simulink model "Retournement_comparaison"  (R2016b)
settings: Solver=ode15s  StartTime=0.0  StopTime=15000  MaxStep=100  RelTol=1e-2  AbsTol=1e-2
undefined symbols (not defined in the file or in its folder): Bague, Bielle, Chassis, deg, kg, m, Manivelle, mm, Moteur, N, Panier_Oeuf, RootGround, RootPart, s, sigbuilder_block, Support_oeufs, Vis
libraries: mblibv1 x42, fl_lib x7, nesl_utility x3, elec_lib x2

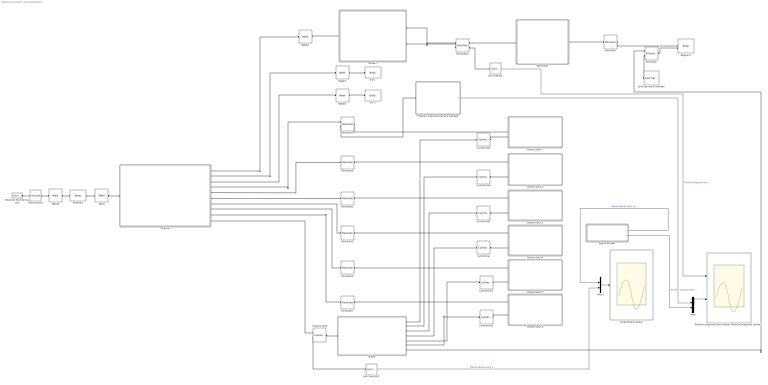
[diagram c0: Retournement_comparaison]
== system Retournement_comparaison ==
  Bague-2 : mblibv1/Bodies/Body  LConnTagsString=CS2|CS3  UpdateFromCAD=on  PMImportedID=Bague-2  DialogClass=MechanicalBodyBlock  Mass=2.57168e-05  MassUnits=kg  InertiaUnits=kg*m^2  Inertia=[4.96681e-11,0,0;0,4.96681e-11,0;0,0,8.21917e-11]  Shape=Cylinder  ShapeDims=[1 1]  ShapeUnits=m  ShapeUse=false  Density=1  DensityUnits=kg/m^3  DensityUse=false  GraphicsMode=GFXFILE  GraphicsFileName=Panier_Oeuf - Bague-2.STL  BodyColorSelMode=COLORPALETTE  BodyColor=[1;0;0]  AttachedToCS=CS1  CG=Right$CG$[0.256568 -0.0741614 -0.063]$WORLD$WORLD$m$[0.897068 0.441893 0;0 0 1;0.441893 -0.897068 0]$3x3 Transform$rad$WORLD$false$Bague-2::CG(AUTOGEN)  WorkingFrames=Right$CS1$[0.256568 -0.0751614 -0.063]$WORLD$WORLD$m$[0.897068 0.441893 0;0 0 1;0.441893 -0.897068 0]$3x3 Transform$rad$WORLD$false$Bague-2::CS1(AUTOGEN)#Left$CS2$[0.256568 -0.0731614 -0.063]$WORLD$WORLD$m$[1 0 0;0 1 0;0 0 1]$3x3 Transform$rad$WORLD$true$Bague-2:-:Manivelle-1::Bague-2(AUTOGEN)#Left$CS3$[0.254568 -0.0731614 -0.065]$WORLD$WORLD$m$[1 0 0;0 1 0;0 0 1]$3x3 Transform$rad$WORLD$true$Bagu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  CGPos=[0.256568 -0.0741614 -0.063]  CGRot=[0.897068 0.441893 0;0 0 1;0.441893 -0.897068 0]  CS0Pos=[]  CS0Rot=[]  CS1Pos=[0.256568 -0.0751614 -0.063]  CS1Rot=[0.897068 0.441893 0;0 0 1;0.441893 -0.897068 0]  CS2Pos=[0.256568 -0.0731614 -0.063]  CS2Rot=[1 0 0;0 1 0;0 0 1]  CS3Pos=[0.254568 -0.0731614 -0.065]  CS3Rot=[1 0 0;0 1 0;0 0 1]  CS4Pos=[]  CS4Rot=[]  CS5Pos=[]  CS5Rot=[]  CS6Pos=[]  CS6Rot=[]  CS7Pos=[]  CS7Rot=[]  CS8Pos=[]  CS8Rot=[]  CS9Pos=[]  CS9Rot=[]  CS10Pos=[]  CS10Rot=[]  CS11Pos=[]  CS11Rot=[]  CS12Pos=[]  CS12Rot=[]  CS13Pos=[]  CS13Rot=[]  CS14Pos=[]  CS14Rot=[]  CS15Pos=[]  CS15Rot=[]  CS16Pos=[]  CS16Rot=[]  CS17Pos=[]  CS17Rot=[]  CS18Pos=[]  CS18Rot=[]  CS19Pos=[]  CS19Rot=[]  CS20Pos=[]  CS20Rot=[]
  Bielle : Subsystem
  Chassis : Subsystem
  "Cinématique bielle " : Scope
  Custom Joint : mblibv1/Joints/Custom Joint  LConnTagsString=__newl0|SA1  RConnTagsString=__newr0  UpdateFromCAD=on  PMImportedID=Bielle-1:-:Chassis-1  NumSAPorts=1  CutJoint=off  MarkAsCut=off  Primitives=prismatic  PrimitiveProps=P1$World$[1,0,0]$prismatic#P2$World$[0,1,0]$prismatic#P3$World$[0,0,1]$prismatic#R1$World$[0,-1,0]$revolute  DialogClass=JointBlock  R1Axis=[0,-1,0]  R2Axis=[]  R3Axis=[]  P1Axis=[1,0,0]  P2Axis=[0,1,0]  P3Axis=[0,0,1]  SAxis=[]
  Cylindrical : mblibv1/Joints/Cylindrical  LConnTagsString=__newl0  RConnTagsString=__newr0  UpdateFromCAD=on  PMImportedID=Bielle-1:-:Support_oeufs-4  NumSAPorts=0  CutJoint=off  MarkAsCut=off  Primitives=prismatic  PrimitiveProps=P1$WORLD$[0,-1,0]$prismatic#R1$WORLD$[0,-1,0]$revolute  DialogClass=JointBlock  P1Axis=[0,-1,0]  R1Axis=[0,-1,0]
  Cylindrical1 : mblibv1/Joints/Cylindrical  LConnTagsString=__newl0  RConnTagsString=__newr0  UpdateFromCAD=on  PMImportedID=Bielle-1:-:Support_oeufs-3  NumSAPorts=0  CutJoint=off  MarkAsCut=off  Primitives=prismatic  PrimitiveProps=P1$WORLD$[0,-1,0]$prismatic#R1$WORLD$[0,-1,0]$revolute  DialogClass=JointBlock  P1Axis=[0,-1,0]  R1Axis=[0,-1,0]
  Cylindrical2 : mblibv1/Joints/Cylindrical  LConnTagsString=__newl0  RConnTagsString=__newr0  UpdateFromCAD=on  PMImportedID=Bielle-1:-:Support_oeufs-5  NumSAPorts=0  CutJoint=off  MarkAsCut=off  Primitives=prismatic  PrimitiveProps=P1$WORLD$[0,-1,0]$prismatic#R1$WORLD$[0,-1,0]$revolute  DialogClass=JointBlock  P1Axis=[0,-1,0]  R1Axis=[0,-1,0]
  Cylindrical3 : mblibv1/Joints/Cylindrical  LConnTagsString=__newl0  RConnTagsString=__newr0  UpdateFromCAD=on  PMImportedID=Bielle-1:-:Support_oeufs-6  NumSAPorts=0  CutJoint=off  MarkAsCut=off  Primitives=prismatic  PrimitiveProps=P1$WORLD$[0,-1,0]$prismatic#R1$WORLD$[0,-1,0]$revolute  DialogClass=JointBlock  P1Axis=[0,-1,0]  R1Axis=[0,-1,0]
  Cylindrical4 : mblibv1/Joints/Cylindrical  LConnTagsString=__newl0  RConnTagsString=__newr0  UpdateFromCAD=on  PMImportedID=Bielle-1:-:Support_oeufs-2  NumSAPorts=0  CutJoint=off  MarkAsCut=off  Primitives=prismatic  PrimitiveProps=P1$WORLD$[0,-1,0]$prismatic#R1$WORLD$[0,-1,0]$revolute  DialogClass=JointBlock  P1Axis=[0,-1,0]  R1Axis=[0,-1,0]
  Cylindrical5 : mblibv1/Joints/Cylindrical  LConnTagsString=__newl0  RConnTagsString=__newr0  UpdateFromCAD=on  PMImportedID=Bielle-1:-:Support_oeufs-1  NumSAPorts=0  CutJoint=off  MarkAsCut=off  Primitives=prismatic  PrimitiveProps=P1$WORLD$[0,-1,0]$prismatic#R1$WORLD$[0,-1,0]$revolute  DialogClass=JointBlock  P1Axis=[0,-1,0]  R1Axis=[0,-1,0]
  Joint Sensor : mblibv1/Sensors &  Actuators/Joint Sensor  UpdateFromCAD=off  PhysicalDomain=Mechanical  PortType=blob  Muxed=off  Pose=off  Angle=on  AngleUnits=deg  ArcVelocity=off  ArcVelocityUnits=rpm  ArcAcceleration=off  ArcAccelerationUnits=deg/s^2  CoordPosition=on  CoordPositionUnits=m  Velocity=off  VelocityUnits=m/s  Acceleration=off  AccelerationUnits=m/s^2  Quaternion=on  QuaternionDT=off  QuaternionDDT=off  QuaternionUnits=off  OutputVector=[1]  ActiveIO=on  Width=1  DialogClass=MechanicalSensorBlock  Primitive=R1  Force=off  ForceUnits=N  Torque=off  TorqueUnits=N*m  ReferenceFrame=Absolute (World)  ReactionSensedSide=Follower  ReactionReferenceFrame=Absolute (World)  ReactionForce=off  ReactionForceUnits=N  ReactionMoment=off  ReactionMomentUnits=N*m
  Joint Sensor3 : mblibv1/Sensors &  Actuators/Joint Sensor  UpdateFromCAD=off  PhysicalDomain=Mechanical  PortType=blob  Muxed=off  Pose=off  Angle=on  AngleUnits=deg  ArcVelocity=off  ArcVelocityUnits=rpm  ArcAcceleration=off  ArcAccelerationUnits=deg/s^2  CoordPosition=on  CoordPositionUnits=mm  Velocity=off  VelocityUnits=mm/s  Acceleration=off  AccelerationUnits=m/s^2  Quaternion=on  QuaternionDT=off  QuaternionDDT=off  QuaternionUnits=off  OutputVector=[1]  ActiveIO=on  Width=1  DialogClass=MechanicalSensorBlock  Primitive=P1  Force=off  ForceUnits=N  Torque=off  TorqueUnits=N*m  ReferenceFrame=Absolute (World)  ReactionSensedSide=Follower  ReactionReferenceFrame=Absolute (World)  ReactionForce=off  ReactionForceUnits=N  ReactionMoment=off  ReactionMomentUnits=N*m
  Joint Spring & Damper : mblibv1/Force  Elements/Joint Spring & Damper  UpdateFromCAD=off  DialogClass=JointSpringDamper  JFEParameters=P1$true$0$0.1$0$m$m/s$N$deg$deg/s$N*m#P2$false$0$0$0$m$m/s$N$deg$deg/s$N*m#P3$false$0$0$0$m$m/s$N$deg$deg/s$N*m#R1$false$0$0$0$m$m/s$N$deg$deg/s$N*m#R2$false$0$0$0$m$m/s$N$deg$deg/s$N*m#R3$false$0$0$0$m$m/s$N$deg$deg/s$N*m#S$false$0$0$0$m$m/s$N$deg$deg/s$N*m
  Machine Environment1 : mblibv1/Bodies/Machine Environment  PortType=env  PhysicalDomain=Mechanical  DialogTemplateClass=MECH.MachineEnvironment  SyncWhenCopied=off  Gravity=[0 -9.81 0]  GravityUnits=m/s^2  GravityAsSignal=off  Dimensionality=Auto-detect  AnalysisType=Forward dynamics  LinearAssemblyTolerance=1e-3  LinearAssemblyToleranceUnits=m  AngularAssemblyTolerance=1e-3  AngularAssemblyToleranceUnits=rad  ConstraintSolverType=Tolerancing  ConstraintRelTolerance=1e-3  ConstraintAbsTolerance=1e-3  UseRobustSingularityHandling=off  RedundancyAnalysisToleranceType=Specify tolerance  RedundancyAnalysisTolerance=1e-5  StatePerturbationType=Fixed  PerturbationSize=1e-5  VisualizeMachine=on  BodyVisualizationType=Use model default body geometries  BodyColorSelMode=Use model default  DefaultBodyColor=[1 0 0]
  Manivelle : Subsystem
  Moteur : Subsystem
  Mux : Mux  Inputs=2
  Mux1 : Mux  Inputs=2
  Panier Oeuf 1 : Subsystem
  Panier Oeuf 2 : Subsystem
  Panier Oeuf 3 : Subsystem
  Panier Oeuf 4 : Subsystem
  Panier Oeuf 5 : Subsystem
  Panier Oeuf 6 : Subsystem
  Position angulaire Paniers simulée : Subsystem
  "Position angulaire axe moteur Position angulaire paniers " : Scope  NumInputPorts=2
  Prismatic : mblibv1/Joints/Prismatic  LConnTagsString=__newl0|SA1  RConnTagsString=__newr0  UpdateFromCAD=on  PMImportedID=Bague-2:-:Bielle-1  NumSAPorts=1  CutJoint=off  MarkAsCut=off  Primitives=prismatic  PrimitiveProps=P1$World$[0,0,1]$prismatic  DialogClass=JointBlock  P1Axis=[0,0,1]
  Revolute : mblibv1/Joints/Revolute  LConnTagsString=__newl0  RConnTagsString=__newr0  UpdateFromCAD=on  PMImportedID=Bague-2:-:Manivelle-1  NumSAPorts=0  CutJoint=off  MarkAsCut=off  Primitives=prismatic  PrimitiveProps=R1$WORLD$[0,1,0]$revolute  DialogClass=JointBlock  R1Axis=[0,1,0]
  Revolute1 : mblibv1/Joints/Revolute  LConnTagsString=__newl0  RConnTagsString=__newr0  UpdateFromCAD=on  PMImportedID=Chassis-1:-:Support_oeufs-4  NumSAPorts=0  CutJoint=off  MarkAsCut=off  Primitives=prismatic  PrimitiveProps=R1$WORLD$[0,-1,0]$revolute  DialogClass=JointBlock  R1Axis=[0,-1,0]
  Revolute2 : mblibv1/Joints/Revolute  LConnTagsString=__newl0  RConnTagsString=__newr0  UpdateFromCAD=on  PMImportedID=Chassis-1:-:Support_oeufs-3  NumSAPorts=0  CutJoint=off  MarkAsCut=off  Primitives=prismatic  PrimitiveProps=R1$WORLD$[0,-1,0]$revolute  DialogClass=JointBlock  R1Axis=[0,-1,0]
  Revolute3 : mblibv1/Joints/Revolute  LConnTagsString=__newl0|SA1  RConnTagsString=__newr0|SA1  UpdateFromCAD=on  PMImportedID=Manivelle-1:-:Moteur-1  NumSAPorts=2  CutJoint=off  MarkAsCut=off  Primitives=prismatic  PrimitiveProps=R1$World$[0,-1,0]$revolute  DialogClass=JointBlock  R1Axis=[0,-1,0]
  Revolute5 : mblibv1/Joints/Revolute  LConnTagsString=__newl0  RConnTagsString=__newr0  UpdateFromCAD=on  PMImportedID=Chassis-1:-:Support_oeufs-5  NumSAPorts=0  CutJoint=off  MarkAsCut=off  Primitives=prismatic  PrimitiveProps=R1$WORLD$[0,-1,0]$revolute  DialogClass=JointBlock  R1Axis=[0,-1,0]
  Revolute7 : mblibv1/Joints/Revolute  LConnTagsString=__newl0  RConnTagsString=__newr0  UpdateFromCAD=on  PMImportedID=Chassis-1:-:Support_oeufs-6  NumSAPorts=0  CutJoint=off  MarkAsCut=off  Primitives=prismatic  PrimitiveProps=R1$WORLD$[0,-1,0]$revolute  DialogClass=JointBlock  R1Axis=[0,-1,0]
  Revolute8 : mblibv1/Joints/Revolute  LConnTagsString=__newl0  RConnTagsString=__newr0  UpdateFromCAD=on  PMImportedID=Chassis-1:-:Support_oeufs-2  NumSAPorts=0  CutJoint=off  MarkAsCut=off  Primitives=prismatic  PrimitiveProps=R1$WORLD$[0,-1,0]$revolute  DialogClass=JointBlock  R1Axis=[0,-1,0]
  Revolute9 : mblibv1/Joints/Revolute  LConnTagsString=__newl0|SA1  RConnTagsString=__newr0  UpdateFromCAD=on  PMImportedID=Chassis-1:-:Support_oeufs-1  NumSAPorts=1  CutJoint=off  MarkAsCut=off  Primitives=prismatic  PrimitiveProps=R1$World$[0,-1,0]$revolute  DialogClass=JointBlock  R1Axis=[0,-1,0]
  RootGround : mblibv1/Bodies/Ground  UpdateFromCAD=on  PMImportedID=RootGround  LeftPortType=env  RightPortType=workingframe  PhysicalDomain=Mechanical  DialogClass=GroundBlock  CoordPosition=[0.0985288,0.0399076,-0.023573]  CoordPositionUnits=m  StateVectorMgrId=-1  MachineId=[0 0]  ShowEnvPort=on  ParameterChecksum=[42814579, 2142450646, 2016383780, 4272844323]  TopologyChecksum=[3713097820, 1283573318, 1879926558, 343871556]
  RootPart : mblibv1/Bodies/Body  LConnTagsString=CS3  RConnTagsString=CS2  UpdateFromCAD=on  PMImportedID=Panier_Oeuf/RootPart  DialogClass=MechanicalBodyBlock  Mass=0  MassUnits=kg  InertiaUnits=kg*m^2  Inertia=[0,0,0;0,0,0;0,0,0]  Shape=Cylinder  ShapeDims=[1 1]  ShapeUnits=m  ShapeUse=false  Density=1  DensityUnits=kg/m^3  DensityUse=false  GraphicsMode=MACHINE_DEFAULT  BodyColorSelMode=MACHINE_DEFAULT  BodyColor=[1;0;0]  AttachedToCS=CS1  CG=Right$CG$[0.0985288 0.0399076 -0.023573]$WORLD$WORLD$m$[1 0 0;0 1 0;0 0 1]$3x3 Transform$rad$WORLD$false$Panier_Oeuf/RootPart::CG(AUTOGEN)  WorkingFrames=Right$CS1$[0 0 0]$WORLD$WORLD$m$[1 0 0;0 1 0;0 0 1]$3x3 Transform$rad$WORLD$false$Panier_Oeuf/RootPart::CS1(AUTOGEN)#Right$CS2$[0.0811984 0.0557636 -0.00887792]$WORLD$WORLD$m$[1 0 0;0 1 0;0 0 1]$3x3 Transform$rad$WORLD$true$Chassis-1:-:Panier_Oeuf/RootPart::Panier_Oeuf/RootPart(AUTOGEN)#Left$CS3$[0.0985288 0.0399076 -0.023573]$WORLD$WORLD$m$[1 0 0;0 1 0;0 0 1]$3x3 Transform$rad$WORLD$true$Panier_O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  CGPos=[0.0985288 0.0399076 -0.023573]  CGRot=[1 0 0;0 1 0;0 0 1]  CS0Pos=[]  CS0Rot=[]  CS1Pos=[0 0 0]  CS1Rot=[1 0 0;0 1 0;0 0 1]  CS2Pos=[0.0811984 0.0557636 -0.00887792]  CS2Rot=[1 0 0;0 1 0;0 0 1]  CS3Pos=[0.0985288 0.0399076 -0.023573]  CS3Rot=[1 0 0;0 1 0;0 0 1]  CS4Pos=[]  CS4Rot=[]  CS5Pos=[]  CS5Rot=[]  CS6Pos=[]  CS6Rot=[]  CS7Pos=[]  CS7Rot=[]  CS8Pos=[]  CS8Rot=[]  CS9Pos=[]  CS9Rot=[]  CS10Pos=[]  CS10Rot=[]  CS11Pos=[]  CS11Rot=[]  CS12Pos=[]  CS12Rot=[]  CS13Pos=[]  CS13Rot=[]  CS14Pos=[]  CS14Rot=[]  CS15Pos=[]  CS15Rot=[]  CS16Pos=[]  CS16Rot=[]  CS17Pos=[]  CS17Rot=[]  CS18Pos=[]  CS18Rot=[]  CS19Pos=[]  CS19Rot=[]  CS20Pos=[]  CS20Rot=[]
  Signal Builder : Subsystem  Tag=STV Subsys  LoadFcn=sigbuilder_block('load');  StartFcn=sigbuilder_block('start');  StopFcn=sigbuilder_block('stop');  ClipboardFcn=sigbuilder_block('clipboard');
  Vis-1 : mblibv1/Bodies/Body  LConnTagsString=CS2  UpdateFromCAD=on  PMImportedID=Vis-1  DialogClass=MechanicalBodyBlock  Mass=0.000201069  MassUnits=kg  InertiaUnits=kg*m^2  Inertia=[1.44008e-09,0,0;0,1.44008e-09,0;0,0,1.17522e-09]  Shape=Cylinder  ShapeDims=[1 1]  ShapeUnits=m  ShapeUse=false  Density=1  DensityUnits=kg/m^3  DensityUse=false  GraphicsMode=GFXFILE  GraphicsFileName=Panier_Oeuf - Vis-1.STL  BodyColorSelMode=COLORPALETTE  BodyColor=[0.792157;0.819608;0.933333]  AttachedToCS=CS1  CG=Right$CG$[0.274549 -0.0683931 -0.022]$WORLD$WORLD$m$[-0.990019 -0.140935 0;0 0 1;-0.140935 0.990019 0]$3x3 Transform$rad$WORLD$false$Vis-1::CG(AUTOGEN)  WorkingFrames=Right$CS1$[0.274549 -0.0681614 -0.022]$WORLD$WORLD$m$[-0.990019 -0.140935 0;0 0 1;-0.140935 0.990019 0]$3x3 Transform$rad$WORLD$false$Vis-1::CS1(AUTOGEN)#Left$CS2$[0.274549 -0.0681614 -0.022]$WORLD$WORLD$m$[1 0 0;0 1 0;0 0 1]$3x3 Transform$rad$WORLD$true$Chassis-1:-:Vis-1::Vis-1(AUTOGEN)  CGPos=[0.274549 -0.0683931 -0.022]  CGRot=[-0.990019 -0.140935 0;0 0 1;-0.140935 0.990019 0]  CS0Pos=[]  CS0Rot=[]  CS1Pos=[0.274549 -0.0681614 -0.022]  CS1Rot=[-0.990019 -0.140935 0;0 0 1;-0.140935 0.990019 0]  CS2Pos=[0.274549 -0.0681614 -0.022]  CS2Rot=[1 0 0;0 1 0;0 0 1]  CS3Pos=[]  CS3Rot=[]  CS4Pos=[]  CS4Rot=[]  CS5Pos=[]  CS5Rot=[]  CS6Pos=[]  CS6Rot=[]  CS7Pos=[]  CS7Rot=[]  CS8Pos=[]  CS8Rot=[]  CS9Pos=[]  CS9Rot=[]  CS10Pos=[]  CS10Rot=[]  CS11Pos=[]  CS11Rot=[]  CS12Pos=[]  CS12Rot=[]  CS13Pos=[]  CS13Rot=[]  CS14Pos=[]  CS14Rot=[]  CS15Pos=[]  CS15Rot=[]  CS16Pos=[]  CS16Rot=[]  CS17Pos=[]  CS17Rot=[]  CS18Pos=[]  CS18Rot=[]  CS19Pos=[]  CS19Rot=[]  CS20Pos=[]  CS20Rot=[]
  Vis-2 : mblibv1/Bodies/Body  LConnTagsString=CS2  UpdateFromCAD=on  PMImportedID=Vis-2  DialogClass=MechanicalBodyBlock  Mass=0.000201069  MassUnits=kg  InertiaUnits=kg*m^2  Inertia=[1.44008e-09,0,0;0,1.44008e-09,0;0,0,1.17522e-09]  Shape=Cylinder  ShapeDims=[1 1]  ShapeUnits=m  ShapeUse=false  Density=1  DensityUnits=kg/m^3  DensityUse=false  GraphicsMode=GFXFILE  GraphicsFileName=Panier_Oeuf - Vis-2.STL  BodyColorSelMode=COLORPALETTE  BodyColor=[0.792157;0.819608;0.933333]  AttachedToCS=CS1  CG=Right$CG$[0.262549 -0.0683931 -0.022]$WORLD$WORLD$m$[-0.990019 -0.140935 0;0 0 1;-0.140935 0.990019 0]$3x3 Transform$rad$WORLD$false$Vis-2::CG(AUTOGEN)  WorkingFrames=Right$CS1$[0.262549 -0.0681614 -0.022]$WORLD$WORLD$m$[-0.990019 -0.140935 0;0 0 1;-0.140935 0.990019 0]$3x3 Transform$rad$WORLD$false$Vis-2::CS1(AUTOGEN)#Left$CS2$[0.262549 -0.0681614 -0.022]$WORLD$WORLD$m$[1 0 0;0 1 0;0 0 1]$3x3 Transform$rad$WORLD$true$Chassis-1:-:Vis-2::Vis-2(AUTOGEN)  CGPos=[0.262549 -0.0683931 -0.022]  CGRot=[-0.990019 -0.140935 0;0 0 1;-0.140935 0.990019 0]  CS0Pos=[]  CS0Rot=[]  CS1Pos=[0.262549 -0.0681614 -0.022]  CS1Rot=[-0.990019 -0.140935 0;0 0 1;-0.140935 0.990019 0]  CS2Pos=[0.262549 -0.0681614 -0.022]  CS2Rot=[1 0 0;0 1 0;0 0 1]  CS3Pos=[]  CS3Rot=[]  CS4Pos=[]  CS4Rot=[]  CS5Pos=[]  CS5Rot=[]  CS6Pos=[]  CS6Rot=[]  CS7Pos=[]  CS7Rot=[]  CS8Pos=[]  CS8Rot=[]  CS9Pos=[]  CS9Rot=[]  CS10Pos=[]  CS10Rot=[]  CS11Pos=[]  CS11Rot=[]  CS12Pos=[]  CS12Rot=[]  CS13Pos=[]  CS13Rot=[]  CS14Pos=[]  CS14Rot=[]  CS15Pos=[]  CS15Rot=[]  CS16Pos=[]  CS16Rot=[]  CS17Pos=[]  CS17Rot=[]  CS18Pos=[]  CS18Rot=[]  CS19Pos=[]  CS19Rot=[]  CS20Pos=[]  CS20Rot=[]
  Weld : mblibv1/Joints/Weld  LConnTagsString=__newl0  RConnTagsString=__newr0  UpdateFromCAD=on  PMImportedID=Chassis-1:-:Panier_Oeuf/RootPart  NumSAPorts=0  CutJoint=off  MarkAsCut=off  Primitives=weld  PrimitiveProps=W$WORLD$[0.57735,0.57735,0.57735]$weld  DialogClass=JointBlock  WAxis=[0.57735,0.57735,0.57735]
  Weld1 : mblibv1/Joints/Weld  LConnTagsString=__newl0  RConnTagsString=__newr0  UpdateFromCAD=on  PMImportedID=Chassis-1:-:Moteur-1  NumSAPorts=0  CutJoint=off  MarkAsCut=off  Primitives=weld  PrimitiveProps=W$WORLD$[0.57735,0.57735,0.57735]$weld  DialogClass=JointBlock  WAxis=[0.57735,0.57735,0.57735]
  Weld2 : mblibv1/Joints/Weld  LConnTagsString=__newl0  RConnTagsString=__newr0  UpdateFromCAD=on  PMImportedID=Panier_Oeuf/RootPart:-:RootGround  NumSAPorts=0  CutJoint=off  MarkAsCut=off  Primitives=weld  PrimitiveProps=W$WORLD$[0.57735,0.57735,0.57735]$weld  DialogClass=JointBlock  WAxis=[0.57735,0.57735,0.57735]
  Weld3 : mblibv1/Joints/Weld  LConnTagsString=__newl0  RConnTagsString=__newr0  UpdateFromCAD=on  NumSAPorts=0  CutJoint=off  MarkAsCut=off  Primitives=weld  PrimitiveProps=W$WORLD$[0.57735,0.57735,0.57735]$weld  DialogClass=JointBlock  WAxis=[0.57735,0.57735,0.57735]
  Weld4 : mblibv1/Joints/Weld  LConnTagsString=__newl0  RConnTagsString=__newr0  UpdateFromCAD=on  NumSAPorts=0  CutJoint=off  MarkAsCut=off  Primitives=weld  PrimitiveProps=W$WORLD$[0.57735,0.57735,0.57735]$weld  DialogClass=JointBlock  WAxis=[0.57735,0.57735,0.57735]
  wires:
  Joint Sensor/1 -> "Position angulaire axe moteur Position angulaire paniers "/1  "Position angulaire axe moteur simulée"
  Joint Sensor3/1 -> Mux1/2  "Position Bielle axe X simulée"
  Signal Builder/2(Position Ang Paniers) -> Mux/2  "Position angulaire Paniers mesurée"
  Mux/1 -> "Position angulaire axe moteur Position angulaire paniers "/2
  Mux1/1 -> "Cinématique bielle "/1
  Signal Builder/1(Position Bielle Axe X) -> Mux1/1  "Position Bielle axe X mesurée"
  Position angulaire Paniers simulée/1(Out1) -> Mux/1
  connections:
  RootPart/RConn1 -- Weld/LConn1
  Revolute/RConn1 -- Bague-2/LConn1
  Prismatic/RConn1 -- Bague-2/LConn2
  Panier Oeuf 4/LConn1 -- Revolute1/RConn1
  Panier Oeuf 4/LConn2 -- Cylindrical/RConn1
  Panier Oeuf 3/LConn1 -- Revolute2/RConn1
  Panier Oeuf 3/LConn2 -- Cylindrical1/RConn1
  Weld4/RConn1 -- Vis-2/LConn1
  Panier Oeuf 5/LConn1 -- Revolute5/RConn1
  Panier Oeuf 5/LConn2 -- Cylindrical2/RConn1
  Weld3/RConn1 -- Vis-1/LConn1
  Panier Oeuf 6/LConn1 -- Revolute7/RConn1
  Panier Oeuf 2/LConn1 -- Revolute8/RConn1
  Revolute9/RConn1 -- Panier Oeuf 1/LConn1
  Cylindrical3/RConn1 -- Panier Oeuf 6/LConn2
  Panier Oeuf 2/LConn2 -- Cylindrical4/RConn1
  Cylindrical5/RConn1 -- Panier Oeuf 1/LConn2
  RootGround/RConn1 -- Weld2/LConn1
  Weld2/RConn1 -- RootPart/LConn1
  Machine Environment1/RConn1 -- RootGround/LConn1
  Joint Spring & Damper/LConn1 -- Prismatic/LConn2
  Moteur/RConn1 -- Revolute3/LConn1
  Weld1/RConn1 -- Moteur/LConn1
  Revolute3/LConn2 -- Moteur/RConn2
  Manivelle/LConn1 -- Revolute3/RConn1
  Manivelle/RConn1 -- Revolute/LConn1
  Prismatic/LConn1 -- Bielle/RConn7
  Bielle/RConn1 -- Cylindrical5/LConn1
  Bielle/RConn2 -- Cylindrical4/LConn1
  Bielle/RConn3 -- Cylindrical1/LConn1
  Bielle/RConn4 -- Cylindrical/LConn1
  Cylindrical2/LConn1 -- Bielle/RConn5
  Bielle/RConn6 -- Cylindrical3/LConn1
  Custom Joint/RConn1 -- Bielle/LConn1
  Weld1/LConn1 -- Chassis/RConn1
  Weld3/LConn1 -- Chassis/RConn2
  Weld4/LConn1 -- Chassis/RConn3
  Revolute9/LConn1 -- Chassis/RConn4
  Revolute8/LConn1 -- Chassis/RConn5
  Revolute2/LConn1 -- Chassis/RConn6
  Revolute1/LConn1 -- Chassis/RConn7
  Weld/RConn1 -- Chassis/LConn1
  Revolute5/LConn1 -- Chassis/RConn8
  Revolute7/LConn1 -- Chassis/RConn9
  Custom Joint/LConn1 -- Chassis/RConn10
  Revolute3/RConn2 -- Joint Sensor/LConn1
  Custom Joint/LConn2 -- Joint Sensor3/LConn1
  Position angulaire Paniers simulée/LConn1 -- Revolute9/LConn2

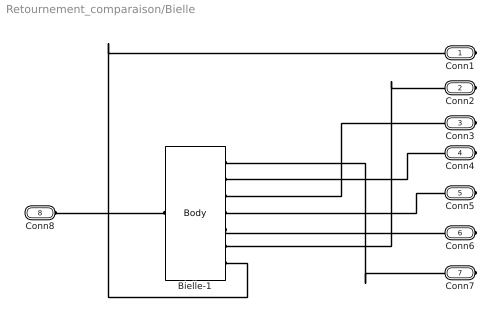
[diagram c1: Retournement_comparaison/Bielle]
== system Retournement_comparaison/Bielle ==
  Bielle-1 : mblibv1/Bodies/Body  LConnTagsString=CS6  RConnTagsString=CS2|CS3|CS4|CS5|CS7|CS8|CS9  UpdateFromCAD=on  PMImportedID=Bielle-1  DialogClass=MechanicalBodyBlock  Mass=0.0183422  MassUnits=kg  InertiaUnits=kg*m^2  Inertia=[1.02402e-06,1.48492e-06,-1.23168e-06;1.48492e-06,0.000206355,2.24204e-08;-1.23168e-06,2.24204e-08,0.00020726]  Shape=Cylinder  ShapeDims=[1 1]  ShapeUnits=m  ShapeUse=false  Density=1  DensityUnits=kg/m^3  DensityUse=false  GraphicsMode=GFXFILE  GraphicsFileName=Panier_Oeuf - Bielle-1.STL  BodyColorSelMode=COLORPALETTE  BodyColor=[1;1;0]  AttachedToCS=CS1  CG=Right$CG$[0.125761 -0.080148 -0.0505953]$WORLD$WORLD$m$[-1 0 0;0 0 -1;0 -1 0]$3x3 Transform$rad$WORLD$false$Bielle-1::CG(AUTOGEN)  WorkingFrames=Right$CS1$[0.231882 -0.0791614 -0.0940911]$WORLD$WORLD$m$[-1 0 0;0 0 -1;0 -1 0]$3x3 Transform$rad$WORLD$false$Bielle-1::CS1(AUTOGEN)#Right$CS2$[0.254568 -0.0731614 -0.0309764]$WORLD$WORLD$m$[1 0 0;0 1 0;0 0 1]$3x3 Transform$rad$WORLD$true$Bague-2:-:Bielle-1::Bielle-1(AUTOGEN)#Right$CS3$[0.100768 -0.0791614 -0.0499764]$WORLD$WORLD$m$[1 0 0;0 1 0;0 0 1]$3x3 Transform$rad$WORLD$true$Bielle-1:-:Suppor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  CGPos=[0.125761 -0.080148 -0.0505953]  CGRot=[-1 0 0;0 0 -1;0 -1 0]  CS0Pos=[]  CS0Rot=[]  CS1Pos=[0.231882 -0.0791614 -0.0940911]  CS1Rot=[-1 0 0;0 0 -1;0 -1 0]  CS2Pos=[0.254568 -0.0731614 -0.0309764]  CS2Rot=[1 0 0;0 1 0;0 0 1]  CS3Pos=[0.100768 -0.0791614 -0.0499764]  CS3Rot=[1 0 0;0 1 0;0 0 1]  CS4Pos=[0.046368 -0.0791614 -0.0499764]  CS4Rot=[1 0 0;0 1 0;0 0 1]  CS5Pos=[0.155168 -0.0791614 -0.0499764]  CS5Rot=[1 0 0;0 1 0;0 0 1]  CS6Pos=[0.104549 -0.0681614 0.003]  CS6Rot=[1 0 0;0 1 0;0 0 1]  CS7Pos=[0.209568 -0.0791614 -0.0499764]  CS7Rot=[1 0 0;0 1 0;0 0 1]  CS8Pos=[-0.00803199 -0.0791614 -0.0499764]  CS8Rot=[1 0 0;0 1 0;0 0 1]  CS9Pos=[-0.062432 -0.0791614 -0.0499764]  CS9Rot=[1 0 0;0 1 0;0 0 1]  CS10Pos=[]  CS10Rot=[]  CS11Pos=[]  CS11Rot=[]  CS12Pos=[]  CS12Rot=[]  CS13Pos=[]  CS13Rot=[]  CS14Pos=[]  CS14Rot=[]  CS15Pos=[]  CS15Rot=[]  CS16Pos=[]  CS16Rot=[]  CS17Pos=[]  CS17Rot=[]  CS18Pos=[]  CS18Rot=[]  CS19Pos=[]  CS19Rot=[]  CS20Pos=[]  CS20Rot=[]
  Conn1 : PMIOPort  Port=1  Side=Right
  Conn2 : PMIOPort  Port=2  Side=Right
  Conn3 : PMIOPort  Port=3  Side=Right
  Conn4 : PMIOPort  Port=4  Side=Right
  Conn5 : PMIOPort  Port=5  Side=Right
  Conn6 : PMIOPort  Port=6  Side=Right
  Conn7 : PMIOPort  Port=7  Side=Right
  Conn8 : PMIOPort  Port=8  Side=Left
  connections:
  Bielle-1/RConn4 -- Conn5/RConn1
  Conn8/RConn1 -- Bielle-1/LConn1
  Bielle-1/RConn7 -- Conn1/RConn1
  Bielle-1/RConn5 -- Conn6/RConn1
  Bielle-1/RConn6 -- Conn2/RConn1
  Bielle-1/RConn1 -- Conn7/RConn1
  Bielle-1/RConn2 -- Conn4/RConn1
  Bielle-1/RConn3 -- Conn3/RConn1

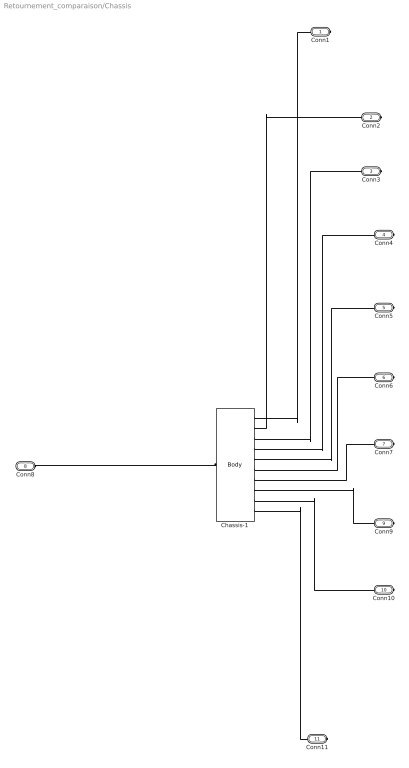
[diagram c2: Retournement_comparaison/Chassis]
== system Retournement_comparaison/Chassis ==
  Chassis-1 : mblibv1/Bodies/Body  LConnTagsString=CS2  RConnTagsString=CS3|CS4|CS5|CS6|CS7|CS8|CS9|CS10|CS11|CS12  UpdateFromCAD=on  PMImportedID=Chassis-1  DialogClass=MechanicalBodyBlock  Mass=0.187115  MassUnits=kg  InertiaUnits=kg*m^2  Inertia=[0.00212227,3.19267e-05,-2.28618e-06;3.19267e-05,0.00278137,7.43577e-06;-2.28618e-06,7.43577e-06,0.00485618]  Shape=Cylinder  ShapeDims=[1 1]  ShapeUnits=m  ShapeUse=false  Density=1  DensityUnits=kg/m^3  DensityUse=false  GraphicsMode=GFXFILE  GraphicsFileName=Panier_Oeuf - Chassis-1.STL  BodyColorSelMode=COLORPALETTE  BodyColor=[0 1 0]  AttachedToCS=CS1  CG=Right$CG$[0.0811984 0.0557636 -0.00887792]$WORLD$WORLD$m$[1 0 0;0 1 0;0 0 1]$3x3 Transform$rad$WORLD$false$Chassis-1::CG(AUTOGEN)  WorkingFrames=Right$CS1$[0 0 0]$WORLD$WORLD$m$[1 0 0;0 1 0;0 0 1]$3x3 Transform$rad$WORLD$false$Chassis-1::CS1(AUTOGEN)#Left$CS2$[0.0811984 0.0557636 -0.00887792]$WORLD$WORLD$m$[1 0 0;0 1 0;0 0 1]$3x3 Transform$rad$WORLD$true$Chassis-1:-:Panier_Oeuf/RootPart::Chassis-1(AUTOGEN)#Right$CS3$[0.282549 -0.0651614 0.003]$WORLD$WORLD$m$[1 0 0;0 1 0;0 0 1]$3x3 Transform$rad$WORLD$true$Chassis-1:-:Support_oeufs-4::Chass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  CGPos=[0.0811984 0.0557636 -0.00887792]  CGRot=[1 0 0;0 1 0;0 0 1]  CS0Pos=[]  CS0Rot=[]  CS1Pos=[0 0 0]  CS1Rot=[1 0 0;0 1 0;0 0 1]  CS2Pos=[0.0811984 0.0557636 -0.00887792]  CS2Rot=[1 0 0;0 1 0;0 0 1]  CS3Pos=[0.282549 -0.0651614 0.003]  CS3Rot=[1 0 0;0 1 0;0 0 1]  CS4Pos=[0.274549 -0.0681614 -0.022]  CS4Rot=[1 0 0;0 1 0;0 0 1]  CS5Pos=[0.262549 -0.0681614 -0.022]  CS5Rot=[1 0 0;0 1 0;0 0 1]  CS6Pos=[-0.0634506 0.192839 -0.028]  CS6Rot=[1 0 0;0 1 0;0 0 1]  CS7Pos=[-0.00905056 -0.0651614 -0.028]  CS7Rot=[1 0 0;0 1 0;0 0 1]  CS8Pos=[0.0453494 0.192839 -0.028]  CS8Rot=[1 0 0;0 1 0;0 0 1]  CS9Pos=[0.0997494 0.192839 -0.028]  CS9Rot=[1 0 0;0 1 0;0 0 1]  CS10Pos=[0.154149 0.192839 -0.028]  CS10Rot=[1 0 0;0 1 0;0 0 1]  CS11Pos=[0.208549 0.192839 -0.028]  CS11Rot=[1 0 0;0 1 0;0 0 1]  CS12Pos=[0.104549 -0.0681614 0.003]  CS12Rot=[1 0 0;0 1 0;0 0 1]  CS13Pos=[]  CS13Rot=[]  CS14Pos=[]  CS14Rot=[]  CS15Pos=[]  CS15Rot=[]  CS16Pos=[]  CS16Rot=[]  CS17Pos=[]  CS17Rot=[]  CS18Pos=[]  CS18Rot=[]  CS19Pos=[]  CS19Rot=[]  CS20Pos=[]  CS20Rot=[]
  Conn1 : PMIOPort  Port=1  Side=Right
  Conn2 : PMIOPort  Port=2  Side=Right
  Conn3 : PMIOPort  Port=3  Side=Right
  Conn4 : PMIOPort  Port=4  Side=Right
  Conn5 : PMIOPort  Port=5  Side=Right
  Conn6 : PMIOPort  Port=6  Side=Right
  Conn7 : PMIOPort  Port=7  Side=Right
  Conn8 : PMIOPort  Port=8  Side=Left
  Conn9 : PMIOPort  Port=9  Side=Right
  Conn10 : PMIOPort  Port=10  Side=Right
  Conn11 : PMIOPort  Port=11  Side=Right
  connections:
  Chassis-1/RConn2 -- Conn2/RConn1
  Conn5/RConn1 -- Chassis-1/RConn5
  Conn10/RConn1 -- Chassis-1/RConn9
  Conn11/RConn1 -- Chassis-1/RConn10
  Conn4/RConn1 -- Chassis-1/RConn4
  Conn7/RConn1 -- Chassis-1/RConn7
  Conn8/RConn1 -- Chassis-1/LConn1
  Conn6/RConn1 -- Chassis-1/RConn6
  Conn1/RConn1 -- Chassis-1/RConn1
  Conn3/RConn1 -- Chassis-1/RConn3
  Conn9/RConn1 -- Chassis-1/RConn8

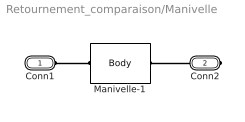
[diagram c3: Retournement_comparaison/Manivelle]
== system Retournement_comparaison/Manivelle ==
  Manivelle-1 : mblibv1/Bodies/Body  LConnTagsString=CS3  RConnTagsString=CS2  UpdateFromCAD=on  DialogClass=MechanicalBodyBlock  Mass=0.00108618  MassUnits=kg  InertiaUnits=kg*m^2  Inertia=[4.74046e-08,2.5744e-14,9.07589e-15;2.5744e-14,1.94685e-08,9.52587e-09;9.07589e-15,9.52587e-09,4.3148e-08]  Shape=Cylinder  ShapeDims=[1 1]  ShapeUnits=m  ShapeUse=false  Density=1  DensityUnits=kg/m^3  DensityUse=false  GraphicsMode=GFXFILE  GraphicsFileName=Panier_Oeuf - Manivelle-1.STL  BodyColorSelMode=COLORPALETTE  BodyColor=[1;0;0]  AttachedToCS=CS1  CG=Right$CG$[0.256553 -0.069861 -0.0518262]$WORLD$WORLD$m$[0.999999 -0.00132653 0;0 0 -1;0.00132653 0.999999 0]$3x3 Transform$rad$WORLD$false$none  WorkingFrames=Right$CS1$[0.256549 -0.0676614 -0.049]$WORLD$WORLD$m$[0.999999 -0.00132653 0;0 0 -1;0.00132653 0.999999 0]$3x3 Transform$rad$WORLD$false$none#Right$CS2$[0.256568 -0.0731614 -0.063]$WORLD$WORLD$m$[1 0 0;0 1 0;0 0 1]$3x3 Transform$rad$WORLD$true$none#Left$CS3$[0.256549 -0.0571614 -0.049]$WORLD$WORLD$m$[1 0 0;0 1 0;0 0 1]$3x3 Transform$rad$WORLD$true$none  CGPos=[0.256553 -0.069861 -0.0518262]  CGRot=[0.999999 -0.00132653 0;0 0 -1;0.00132653 0.999999 0]  CS0Pos=[]  CS0Rot=[]  CS1Pos=[0.256549 -0.0676614 -0.049]  CS1Rot=[0.999999 -0.00132653 0;0 0 -1;0.00132653 0.999999 0]  CS2Pos=[0.256568 -0.0731614 -0.063]  CS2Rot=[1 0 0;0 1 0;0 0 1]  CS3Pos=[0.256549 -0.0571614 -0.049]  CS3Rot=[1 0 0;0 1 0;0 0 1]  CS4Pos=[]  CS4Rot=[]  CS5Pos=[]  CS5Rot=[]  CS6Pos=[]  CS6Rot=[]  CS7Pos=[]  CS7Rot=[]  CS8Pos=[]  CS8Rot=[]  CS9Pos=[]  CS9Rot=[]  CS10Pos=[]  CS10Rot=[]  CS11Pos=[]  CS11Rot=[]  CS12Pos=[]  CS12Rot=[]  CS13Pos=[]  CS13Rot=[]  CS14Pos=[]  CS14Rot=[]  CS15Pos=[]  CS15Rot=[]  CS16Pos=[]  CS16Rot=[]  CS17Pos=[]  CS17Rot=[]  CS18Pos=[]  CS18Rot=[]  CS19Pos=[]  CS19Rot=[]  CS20Pos=[]  CS20Rot=[]
  Conn1 : PMIOPort  Port=1  Side=Left
  Conn2 : PMIOPort  Port=2  Side=Right
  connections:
  Manivelle-1/LConn1 -- Conn1/RConn1
  Manivelle-1/RConn1 -- Conn2/RConn1

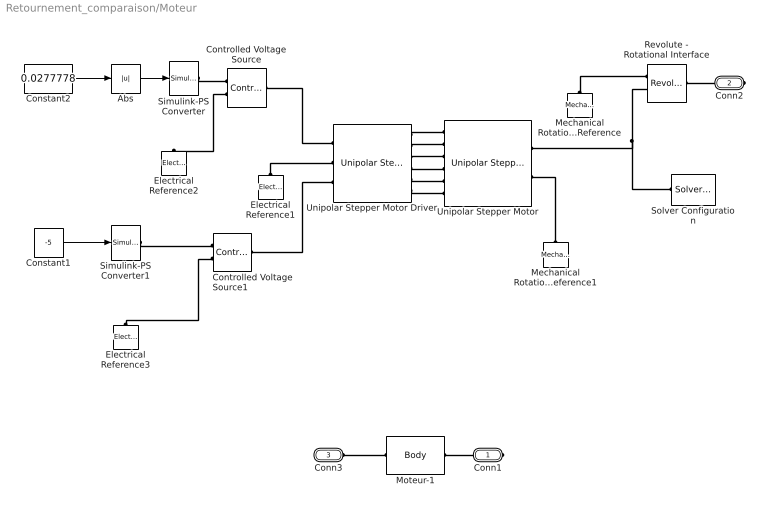
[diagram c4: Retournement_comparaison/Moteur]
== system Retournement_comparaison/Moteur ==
  Abs : Abs
  Constant1 : Constant  Value=-5
  Constant2 : Constant  Value=0.0277778
  Controlled Voltage Source : fl_lib/Electrical/Electrical Sources/Controlled Voltage Source
  Controlled Voltage Source1 : fl_lib/Electrical/Electrical Sources/Controlled Voltage Source
  Electrical Reference1 : fl_lib/Electrical/Electrical Elements/Electrical Reference
  Electrical Reference2 : fl_lib/Electrical/Electrical Elements/Electrical Reference
  Electrical Reference3 : fl_lib/Electrical/Electrical Elements/Electrical Reference
  Mechanical Rotational Reference : fl_lib/Mechanical/Rotational Elements/Mechanical Rotational Reference
  Mechanical Rotational Reference1 : fl_lib/Mechanical/Rotational Elements/Mechanical Rotational Reference
  Moteur-1 : mblibv1/Bodies/Body  LConnTagsString=CS3  RConnTagsString=CS2  UpdateFromCAD=on  DialogClass=MechanicalBodyBlock  Mass=0.0504586  MassUnits=kg  InertiaUnits=kg*m^2  Inertia=[1.06118e-05,4.49291e-11,-3.8172e-09;4.49291e-11,1.05148e-05,4.64072e-08;-3.8172e-09,4.64072e-08,1.45316e-05]  Shape=Cylinder  ShapeDims=[1 1]  ShapeUnits=m  ShapeUse=false  Density=1  DensityUnits=kg/m^3  DensityUse=false  GraphicsMode=GFXFILE  GraphicsFileName=Panier_Oeuf - Moteur-1.STL  BodyColorSelMode=COLORPALETTE  BodyColor=[0.752941;0.752941;0.752941]  AttachedToCS=CS1  CG=Right$CG$[0.268562 -0.0512767 -0.0489313]$WORLD$WORLD$m$[-1 0 0;0 0 -1;0 -1 0]$3x3 Transform$rad$WORLD$false$none  WorkingFrames=Right$CS1$[0.268549 -0.0371614 -0.049]$WORLD$WORLD$m$[-1 0 0;0 0 -1;0 -1 0]$3x3 Transform$rad$WORLD$false$none#Right$CS2$[0.256549 -0.0571614 -0.049]$WORLD$WORLD$m$[1 0 0;0 1 0;0 0 1]$3x3 Transform$rad$WORLD$true$none#Left$CS3$[0.282549 -0.0651614 0.003]$WORLD$WORLD$m$[1 0 0;0 1 0;0 0 1]$3x3 Transform$rad$WORLD$true$none  CGPos=[0.268562 -0.0512767 -0.0489313]  CGRot=[-1 0 0;0 0 -1;0 -1 0]  CS0Pos=[]  CS0Rot=[]  CS1Pos=[0.268549 -0.0371614 -0.049]  CS1Rot=[-1 0 0;0 0 -1;0 -1 0]  CS2Pos=[0.256549 -0.0571614 -0.049]  CS2Rot=[1 0 0;0 1 0;0 0 1]  CS3Pos=[0.282549 -0.0651614 0.003]  CS3Rot=[1 0 0;0 1 0;0 0 1]  CS4Pos=[]  CS4Rot=[]  CS5Pos=[]  CS5Rot=[]  CS6Pos=[]  CS6Rot=[]  CS7Pos=[]  CS7Rot=[]  CS8Pos=[]  CS8Rot=[]  CS9Pos=[]  CS9Rot=[]  CS10Pos=[]  CS10Rot=[]  CS11Pos=[]  CS11Rot=[]  CS12Pos=[]  CS12Rot=[]  CS13Pos=[]  CS13Rot=[]  CS14Pos=[]  CS14Rot=[]  CS15Pos=[]  CS15Rot=[]  CS16Pos=[]  CS16Rot=[]  CS17Pos=[]  CS17Rot=[]  CS18Pos=[]  CS18Rot=[]  CS19Pos=[]  CS19Rot=[]  CS20Pos=[]  CS20Rot=[]
  Revolute - Rotational Interface : mblibv1/Interface  Elements/Revolute - Rotational Interface  UpdateFromCAD=off  DialogClass=RevoluteRotationalInterface  Primitive=R1  InputFiltering=on  SimscapeFilterOrder=1  InputFilterTimeConstant=0.001
  Simulink-PS Converter : nesl_utility/Simulink-PS Converter  PhysicalDomain=network_engine_domain  SubClassName=ps_input  LeftPortType=input  RightPortType=output  PseudoPeriodic=off  Frequencies=[]  NoiseDistribution=none  NoiseParameters=[]  Unit=1  AffineConversion=off  InputFiltering=off  SimscapeFilterOrder=1  InputFilterTimeConstant=0.001  UdotUserProvided=1
  Simulink-PS Converter1 : nesl_utility/Simulink-PS Converter  PhysicalDomain=network_engine_domain  SubClassName=ps_input  LeftPortType=input  RightPortType=output  PseudoPeriodic=off  Frequencies=[]  NoiseDistribution=none  NoiseParameters=[]  Unit=V  AffineConversion=off  InputFiltering=off  SimscapeFilterOrder=1  InputFilterTimeConstant=0.001  UdotUserProvided=1
  Solver Configuration : nesl_utility/Solver Configuration  PhysicalDomain=network_engine_domain  SubClassName=solver  LeftPortType=input  RightPortType=generic  Accelerate=off  Tones=[]  Harmonics=[]  SimulateNoise=off  Profile=off  UseLocalSampling=off  EnableSwitchedLinearOptims=on  FrequencyDomain=off  UseCCode=off  RelTol=0.001  AbsTol=1e-06  MinStep=1e-09  ToWorkspace=off  RevertToSquareIcSolve=off  NumHomotopyIterations=100  PhasorMode=off  PhasorModeNumHarmonics=1  OverrideAbsTol=off  DoDC=off  ResidualTolerance=1e-09  UseLocalSolver=off  LocalSolverChoice=NE_BACKWARD_EULER_ADVANCER  LocalSolverSampleTime=0.001  DoFixedCost=off  MaxNonlinIter=3  MaxModeIter=2  LinearAlgebra=Sparse  DelaysMemoryBudget=1024  AutomaticFiltering=on  FilteringTimeConstant=0.001
  Unipolar Stepper Motor : elec_lib/Actuators & Drivers/Rotational Actuators/Unipolar Stepper Motor  step_or_av=2  w_vec=[ 0 0.5 1 ] rpm  T_vec=[ 12.2 12.2 11 ] N*m  assert_if_slipping=1  J_total=2+1e-3 kg*m^2  max_step_rate=1 Hz  Ra=0.55 Ohm  La=0.0015 H  Km=0.19 N*m/A  Td=0 N*m  Rm=Inf Ohm  Step=0.9 deg  J=1e-3 kg*m^2  B=1e-3 N*m/(rad/s)  speed0=0 rpm  theta0=-0.9 deg  alpha=0.00393 1/K  Tmeas=25 C  T_vec2=[ 1.7 1.7 0.85 ] N*m  Tmeas2=125 C  half_stepping=0  thermal_mass=100 J/K  initial_temperatures=[ 25 25 25 25 ] C  rotor_thermal_mass=50 J/K  rotor_initial_temperature=25 C  Rm_percent_rotor=90
  Unipolar Stepper Motor Driver : elec_lib/Actuators & Drivers/Drivers/Unipolar Stepper Motor Driver  step_or_av=2  step_rate_per_volt=1 Hz/V  Venable=2.5 V  Vreverse=2.5 V  Vm=5 V  half_stepping=0
  Conn1 : PMIOPort  Port=1  Side=Right
  Conn2 : PMIOPort  Port=2  Side=Right
  Conn3 : PMIOPort  Port=3  Side=Left
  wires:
  Abs/1 -> Simulink-PS Converter/1
  Constant1/1 -> Simulink-PS Converter1/1
  Constant2/1 -> Abs/1
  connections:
  Simulink-PS Converter/RConn1 -- Controlled Voltage Source/RConn1
  Unipolar Stepper Motor Driver/RConn4 -- Unipolar Stepper Motor/LConn4
  Mechanical Rotational Reference/LConn1 -- Revolute - Rotational Interface/LConn1
  Unipolar Stepper Motor Driver/RConn2 -- Unipolar Stepper Motor/LConn2
  Solver Configuration/RConn1 -- Revolute - Rotational Interface/LConn2 -- Unipolar Stepper Motor/RConn1
  Simulink-PS Converter1/RConn1 -- Controlled Voltage Source1/RConn1
  Controlled Voltage Source/LConn1 -- Unipolar Stepper Motor Driver/LConn1
  Revolute - Rotational Interface/RConn1 -- Conn2/RConn1
  Unipolar Stepper Motor Driver/RConn6 -- Unipolar Stepper Motor/LConn6
  Unipolar Stepper Motor Driver/RConn5 -- Unipolar Stepper Motor/LConn5
  Mechanical Rotational Reference1/LConn1 -- Unipolar Stepper Motor/RConn2
  Unipolar Stepper Motor Driver/RConn3 -- Unipolar Stepper Motor/LConn3
  Electrical Reference1/LConn1 -- Unipolar Stepper Motor Driver/LConn2
  Electrical Reference2/LConn1 -- Controlled Voltage Source/RConn2
  Unipolar Stepper Motor Driver/RConn1 -- Unipolar Stepper Motor/LConn1
  Electrical Reference3/LConn1 -- Controlled Voltage Source1/RConn2
  Controlled Voltage Source1/LConn1 -- Unipolar Stepper Motor Driver/LConn3
  Moteur-1/LConn1 -- Conn3/RConn1
  Moteur-1/RConn1 -- Conn1/RConn1

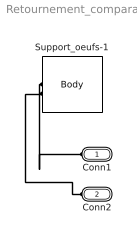
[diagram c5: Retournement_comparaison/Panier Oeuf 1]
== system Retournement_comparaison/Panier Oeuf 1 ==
  Support_oeufs-1 : mblibv1/Bodies/Body  LConnTagsString=CS2|CS3  UpdateFromCAD=on  DialogClass=MechanicalBodyBlock  Mass=0.038981  MassUnits=kg  InertiaUnits=kg*m^2  Inertia=[0.000250911,5.885e-12,5.23692e-11;5.885e-12,0.00026314,-1.7424e-06;5.23692e-11,-1.7424e-06,1.47192e-05]  Shape=Cylinder  ShapeDims=[1 1]  ShapeUnits=m  ShapeUse=false  Density=1  DensityUnits=kg/m^3  DensityUse=false  GraphicsMode=GFXFILE  GraphicsFileName=Panier_Oeuf - Support_oeufs-1.STL  BodyColorSelMode=COLORPALETTE  BodyColor=[1;1;1]  AttachedToCS=CS1  CG=Right$CG$[-0.0634688 0.0570183 -0.0276067]$WORLD$WORLD$m$[-0.998928 -0.0462987 0;0 0 1;-0.0462987 0.998928 0]$3x3 Transform$rad$WORLD$false$none  WorkingFrames=Right$CS1$[-0.0630339 0.0598386 -0.0369903]$WORLD$WORLD$m$[-0.998928 -0.0462987 0;0 0 1;-0.0462987 0.998928 0]$3x3 Transform$rad$WORLD$false$none#Left$CS2$[-0.0634506 0.192839 -0.028]$WORLD$WORLD$m$[1 0 0;0 1 0;0 0 1]$3x3 Transform$rad$WORLD$true$none#Left$CS3$[-0.062432 -0.0791614 -0.0499764]$WORLD$WORLD$m$[1 0 0;0 1 0;0 0 1]$3x3 Transform$rad$WORLD$true$none  CGPos=[-0.0634688 0.0570183 -0.0276067]  CGRot=[-0.998928 -0.0462987 0;0 0 1;-0.0462987 0.998928 0]  CS0Pos=[]  CS0Rot=[]  CS1Pos=[-0.0630339 0.0598386 -0.0369903]  CS1Rot=[-0.998928 -0.0462987 0;0 0 1;-0.0462987 0.998928 0]  CS2Pos=[-0.0634506 0.192839 -0.028]  CS2Rot=[1 0 0;0 1 0;0 0 1]  CS3Pos=[-0.062432 -0.0791614 -0.0499764]  CS3Rot=[1 0 0;0 1 0;0 0 1]  CS4Pos=[]  CS4Rot=[]  CS5Pos=[]  CS5Rot=[]  CS6Pos=[]  CS6Rot=[]  CS7Pos=[]  CS7Rot=[]  CS8Pos=[]  CS8Rot=[]  CS9Pos=[]  CS9Rot=[]  CS10Pos=[]  CS10Rot=[]  CS11Pos=[]  CS11Rot=[]  CS12Pos=[]  CS12Rot=[]  CS13Pos=[]  CS13Rot=[]  CS14Pos=[]  CS14Rot=[]  CS15Pos=[]  CS15Rot=[]  CS16Pos=[]  CS16Rot=[]  CS17Pos=[]  CS17Rot=[]  CS18Pos=[]  CS18Rot=[]  CS19Pos=[]  CS19Rot=[]  CS20Pos=[]  CS20Rot=[]
  Conn1 : PMIOPort  Port=1  Side=Left
  Conn2 : PMIOPort  Port=2  Side=Left
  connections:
  Support_oeufs-1/LConn2 -- Conn2/RConn1
  Support_oeufs-1/LConn1 -- Conn1/RConn1

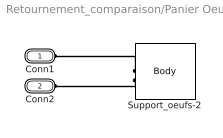
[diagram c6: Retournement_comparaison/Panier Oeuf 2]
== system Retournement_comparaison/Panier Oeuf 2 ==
  Support_oeufs-2 : mblibv1/Bodies/Body  LConnTagsString=CS2|CS3  UpdateFromCAD=on  DialogClass=MechanicalBodyBlock  Mass=0.038981  MassUnits=kg  InertiaUnits=kg*m^2  Inertia=[0.000250911,5.885e-12,5.23692e-11;5.885e-12,0.00026314,-1.7424e-06;5.23692e-11,-1.7424e-06,1.47192e-05]  Shape=Cylinder  ShapeDims=[1 1]  ShapeUnits=m  ShapeUse=false  Density=1  DensityUnits=kg/m^3  DensityUse=false  GraphicsMode=GFXFILE  GraphicsFileName=Panier_Oeuf - Support_oeufs-2.STL  BodyColorSelMode=COLORPALETTE  BodyColor=[1;1;1]  AttachedToCS=CS1  CG=Right$CG$[-0.0090688 0.0570183 -0.0276067]$WORLD$WORLD$m$[-0.998928 -0.0462987 0;0 0 1;-0.0462987 0.998928 0]$3x3 Transform$rad$WORLD$false$none  WorkingFrames=Right$CS1$[-0.00863388 0.0598386 -0.0369903]$WORLD$WORLD$m$[-0.998928 -0.0462987 0;0 0 1;-0.0462987 0.998928 0]$3x3 Transform$rad$WORLD$false$none#Left$CS2$[-0.00905056 -0.0651614 -0.028]$WORLD$WORLD$m$[1 0 0;0 1 0;0 0 1]$3x3 Transform$rad$WORLD$true$none#Left$CS3$[-0.00803199 -0.0791614 -0.0499764]$WORLD$WORLD$m$[1 0 0;0 1 0;0 0 1]$3x3 Transform$rad$WORLD$true$none  CGPos=[-0.0090688 0.0570183 -0.0276067]  CGRot=[-0.998928 -0.0462987 0;0 0 1;-0.0462987 0.998928 0]  CS0Pos=[]  CS0Rot=[]  CS1Pos=[-0.00863388 0.0598386 -0.0369903]  CS1Rot=[-0.998928 -0.0462987 0;0 0 1;-0.0462987 0.998928 0]  CS2Pos=[-0.00905056 -0.0651614 -0.028]  CS2Rot=[1 0 0;0 1 0;0 0 1]  CS3Pos=[-0.00803199 -0.0791614 -0.0499764]  CS3Rot=[1 0 0;0 1 0;0 0 1]  CS4Pos=[]  CS4Rot=[]  CS5Pos=[]  CS5Rot=[]  CS6Pos=[]  CS6Rot=[]  CS7Pos=[]  CS7Rot=[]  CS8Pos=[]  CS8Rot=[]  CS9Pos=[]  CS9Rot=[]  CS10Pos=[]  CS10Rot=[]  CS11Pos=[]  CS11Rot=[]  CS12Pos=[]  CS12Rot=[]  CS13Pos=[]  CS13Rot=[]  CS14Pos=[]  CS14Rot=[]  CS15Pos=[]  CS15Rot=[]  CS16Pos=[]  CS16Rot=[]  CS17Pos=[]  CS17Rot=[]  CS18Pos=[]  CS18Rot=[]  CS19Pos=[]  CS19Rot=[]  CS20Pos=[]  CS20Rot=[]
  Conn1 : PMIOPort  Port=1  Side=Left
  Conn2 : PMIOPort  Port=2  Side=Left
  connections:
  Support_oeufs-2/LConn1 -- Conn1/RConn1
  Support_oeufs-2/LConn2 -- Conn2/RConn1

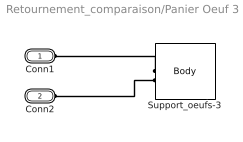
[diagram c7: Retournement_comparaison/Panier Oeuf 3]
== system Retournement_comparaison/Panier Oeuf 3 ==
  Support_oeufs-3 : mblibv1/Bodies/Body  LConnTagsString=CS2|CS3  UpdateFromCAD=on  DialogClass=MechanicalBodyBlock  Mass=0.038981  MassUnits=kg  InertiaUnits=kg*m^2  Inertia=[0.000250911,5.885e-12,5.23692e-11;5.885e-12,0.00026314,-1.7424e-06;5.23692e-11,-1.7424e-06,1.47192e-05]  Shape=Cylinder  ShapeDims=[1 1]  ShapeUnits=m  ShapeUse=false  Density=1  DensityUnits=kg/m^3  DensityUse=false  GraphicsMode=GFXFILE  GraphicsFileName=Panier_Oeuf - Support_oeufs-3.STL  BodyColorSelMode=COLORPALETTE  BodyColor=[1;1;1]  AttachedToCS=CS1  CG=Right$CG$[0.0453312 0.0570183 -0.0276067]$WORLD$WORLD$m$[-0.998928 -0.0462987 0;0 0 1;-0.0462987 0.998928 0]$3x3 Transform$rad$WORLD$false$none  WorkingFrames=Right$CS1$[0.0457661 0.0598386 -0.0369903]$WORLD$WORLD$m$[-0.998928 -0.0462987 0;0 0 1;-0.0462987 0.998928 0]$3x3 Transform$rad$WORLD$false$none#Left$CS2$[0.0453494 0.192839 -0.028]$WORLD$WORLD$m$[1 0 0;0 1 0;0 0 1]$3x3 Transform$rad$WORLD$true$none#Left$CS3$[0.046368 -0.0791614 -0.0499764]$WORLD$WORLD$m$[1 0 0;0 1 0;0 0 1]$3x3 Transform$rad$WORLD$true$none  CGPos=[0.0453312 0.0570183 -0.0276067]  CGRot=[-0.998928 -0.0462987 0;0 0 1;-0.0462987 0.998928 0]  CS0Pos=[]  CS0Rot=[]  CS1Pos=[0.0457661 0.0598386 -0.0369903]  CS1Rot=[-0.998928 -0.0462987 0;0 0 1;-0.0462987 0.998928 0]  CS2Pos=[0.0453494 0.192839 -0.028]  CS2Rot=[1 0 0;0 1 0;0 0 1]  CS3Pos=[0.046368 -0.0791614 -0.0499764]  CS3Rot=[1 0 0;0 1 0;0 0 1]  CS4Pos=[]  CS4Rot=[]  CS5Pos=[]  CS5Rot=[]  CS6Pos=[]  CS6Rot=[]  CS7Pos=[]  CS7Rot=[]  CS8Pos=[]  CS8Rot=[]  CS9Pos=[]  CS9Rot=[]  CS10Pos=[]  CS10Rot=[]  CS11Pos=[]  CS11Rot=[]  CS12Pos=[]  CS12Rot=[]  CS13Pos=[]  CS13Rot=[]  CS14Pos=[]  CS14Rot=[]  CS15Pos=[]  CS15Rot=[]  CS16Pos=[]  CS16Rot=[]  CS17Pos=[]  CS17Rot=[]  CS18Pos=[]  CS18Rot=[]  CS19Pos=[]  CS19Rot=[]  CS20Pos=[]  CS20Rot=[]
  Conn1 : PMIOPort  Port=1  Side=Left
  Conn2 : PMIOPort  Port=2  Side=Left
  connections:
  Support_oeufs-3/LConn2 -- Conn2/RConn1
  Support_oeufs-3/LConn1 -- Conn1/RConn1

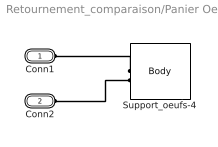
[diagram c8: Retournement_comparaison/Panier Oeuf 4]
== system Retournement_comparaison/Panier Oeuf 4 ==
  Support_oeufs-4 : mblibv1/Bodies/Body  LConnTagsString=CS2|CS3  UpdateFromCAD=on  DialogClass=MechanicalBodyBlock  Mass=0.038981  MassUnits=kg  InertiaUnits=kg*m^2  Inertia=[0.000250911,5.885e-12,5.23692e-11;5.885e-12,0.00026314,-1.7424e-06;5.23692e-11,-1.7424e-06,1.47192e-05]  Shape=Cylinder  ShapeDims=[1 1]  ShapeUnits=m  ShapeUse=false  Density=1  DensityUnits=kg/m^3  DensityUse=false  GraphicsMode=GFXFILE  GraphicsFileName=Panier_Oeuf - Support_oeufs-4.STL  BodyColorSelMode=COLORPALETTE  BodyColor=[1;1;1]  AttachedToCS=CS1  CG=Right$CG$[0.0997312 0.0570183 -0.0276067]$WORLD$WORLD$m$[-0.998928 -0.0462987 0;0 0 1;-0.0462987 0.998928 0]$3x3 Transform$rad$WORLD$false$none  WorkingFrames=Right$CS1$[0.100166 0.0598386 -0.0369903]$WORLD$WORLD$m$[-0.998928 -0.0462987 0;0 0 1;-0.0462987 0.998928 0]$3x3 Transform$rad$WORLD$false$none#Left$CS2$[0.0997494 0.192839 -0.028]$WORLD$WORLD$m$[1 0 0;0 1 0;0 0 1]$3x3 Transform$rad$WORLD$true$none#Left$CS3$[0.100768 -0.0791614 -0.0499764]$WORLD$WORLD$m$[1 0 0;0 1 0;0 0 1]$3x3 Transform$rad$WORLD$true$none  CGPos=[0.0997312 0.0570183 -0.0276067]  CGRot=[-0.998928 -0.0462987 0;0 0 1;-0.0462987 0.998928 0]  CS0Pos=[]  CS0Rot=[]  CS1Pos=[0.100166 0.0598386 -0.0369903]  CS1Rot=[-0.998928 -0.0462987 0;0 0 1;-0.0462987 0.998928 0]  CS2Pos=[0.0997494 0.192839 -0.028]  CS2Rot=[1 0 0;0 1 0;0 0 1]  CS3Pos=[0.100768 -0.0791614 -0.0499764]  CS3Rot=[1 0 0;0 1 0;0 0 1]  CS4Pos=[]  CS4Rot=[]  CS5Pos=[]  CS5Rot=[]  CS6Pos=[]  CS6Rot=[]  CS7Pos=[]  CS7Rot=[]  CS8Pos=[]  CS8Rot=[]  CS9Pos=[]  CS9Rot=[]  CS10Pos=[]  CS10Rot=[]  CS11Pos=[]  CS11Rot=[]  CS12Pos=[]  CS12Rot=[]  CS13Pos=[]  CS13Rot=[]  CS14Pos=[]  CS14Rot=[]  CS15Pos=[]  CS15Rot=[]  CS16Pos=[]  CS16Rot=[]  CS17Pos=[]  CS17Rot=[]  CS18Pos=[]  CS18Rot=[]  CS19Pos=[]  CS19Rot=[]  CS20Pos=[]  CS20Rot=[]
  Conn1 : PMIOPort  Port=1  Side=Left
  Conn2 : PMIOPort  Port=2  Side=Left
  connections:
  Support_oeufs-4/LConn1 -- Conn1/RConn1
  Support_oeufs-4/LConn2 -- Conn2/RConn1

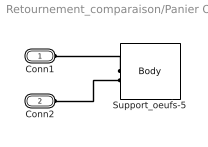
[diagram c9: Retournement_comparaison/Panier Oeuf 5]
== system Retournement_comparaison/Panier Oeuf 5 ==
  Support_oeufs-5 : mblibv1/Bodies/Body  LConnTagsString=CS2|CS3  UpdateFromCAD=on  DialogClass=MechanicalBodyBlock  Mass=0.038981  MassUnits=kg  InertiaUnits=kg*m^2  Inertia=[0.000250911,5.885e-12,5.23692e-11;5.885e-12,0.00026314,-1.7424e-06;5.23692e-11,-1.7424e-06,1.47192e-05]  Shape=Cylinder  ShapeDims=[1 1]  ShapeUnits=m  ShapeUse=false  Density=1  DensityUnits=kg/m^3  DensityUse=false  GraphicsMode=GFXFILE  GraphicsFileName=Panier_Oeuf - Support_oeufs-5.STL  BodyColorSelMode=COLORPALETTE  BodyColor=[1;1;1]  AttachedToCS=CS1  CG=Right$CG$[0.154131 0.0570183 -0.0276067]$WORLD$WORLD$m$[-0.998928 -0.0462987 0;0 0 1;-0.0462987 0.998928 0]$3x3 Transform$rad$WORLD$false$none  WorkingFrames=Right$CS1$[0.154566 0.0598386 -0.0369903]$WORLD$WORLD$m$[-0.998928 -0.0462987 0;0 0 1;-0.0462987 0.998928 0]$3x3 Transform$rad$WORLD$false$none#Left$CS2$[0.154149 0.192839 -0.028]$WORLD$WORLD$m$[1 0 0;0 1 0;0 0 1]$3x3 Transform$rad$WORLD$true$none#Left$CS3$[0.155168 -0.0791614 -0.0499764]$WORLD$WORLD$m$[1 0 0;0 1 0;0 0 1]$3x3 Transform$rad$WORLD$true$none  CGPos=[0.154131 0.0570183 -0.0276067]  CGRot=[-0.998928 -0.0462987 0;0 0 1;-0.0462987 0.998928 0]  CS0Pos=[]  CS0Rot=[]  CS1Pos=[0.154566 0.0598386 -0.0369903]  CS1Rot=[-0.998928 -0.0462987 0;0 0 1;-0.0462987 0.998928 0]  CS2Pos=[0.154149 0.192839 -0.028]  CS2Rot=[1 0 0;0 1 0;0 0 1]  CS3Pos=[0.155168 -0.0791614 -0.0499764]  CS3Rot=[1 0 0;0 1 0;0 0 1]  CS4Pos=[]  CS4Rot=[]  CS5Pos=[]  CS5Rot=[]  CS6Pos=[]  CS6Rot=[]  CS7Pos=[]  CS7Rot=[]  CS8Pos=[]  CS8Rot=[]  CS9Pos=[]  CS9Rot=[]  CS10Pos=[]  CS10Rot=[]  CS11Pos=[]  CS11Rot=[]  CS12Pos=[]  CS12Rot=[]  CS13Pos=[]  CS13Rot=[]  CS14Pos=[]  CS14Rot=[]  CS15Pos=[]  CS15Rot=[]  CS16Pos=[]  CS16Rot=[]  CS17Pos=[]  CS17Rot=[]  CS18Pos=[]  CS18Rot=[]  CS19Pos=[]  CS19Rot=[]  CS20Pos=[]  CS20Rot=[]
  Conn1 : PMIOPort  Port=1  Side=Left
  Conn2 : PMIOPort  Port=2  Side=Left
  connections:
  Support_oeufs-5/LConn1 -- Conn1/RConn1
  Support_oeufs-5/LConn2 -- Conn2/RConn1

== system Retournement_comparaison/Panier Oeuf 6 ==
  Support_oeufs-6 : mblibv1/Bodies/Body  LConnTagsString=CS2|CS3  UpdateFromCAD=on  DialogClass=MechanicalBodyBlock  Mass=0.038981  MassUnits=kg  InertiaUnits=kg*m^2  Inertia=[0.000250911,5.885e-12,5.23692e-11;5.885e-12,0.00026314,-1.7424e-06;5.23692e-11,-1.7424e-06,1.47192e-05]  Shape=Cylinder  ShapeDims=[1 1]  ShapeUnits=m  ShapeUse=false  Density=1  DensityUnits=kg/m^3  DensityUse=false  GraphicsMode=GFXFILE  GraphicsFileName=Panier_Oeuf - Support_oeufs-6.STL  BodyColorSelMode=COLORPALETTE  BodyColor=[1;1;1]  AttachedToCS=CS1  CG=Right$CG$[0.208531 0.0570183 -0.0276067]$WORLD$WORLD$m$[-0.998928 -0.0462987 0;0 0 1;-0.0462987 0.998928 0]$3x3 Transform$rad$WORLD$false$none  WorkingFrames=Right$CS1$[0.208966 0.0598386 -0.0369903]$WORLD$WORLD$m$[-0.998928 -0.0462987 0;0 0 1;-0.0462987 0.998928 0]$3x3 Transform$rad$WORLD$false$none#Left$CS2$[0.208549 0.192839 -0.028]$WORLD$WORLD$m$[1 0 0;0 1 0;0 0 1]$3x3 Transform$rad$WORLD$true$none#Left$CS3$[0.209568 -0.0791614 -0.0499764]$WORLD$WORLD$m$[1 0 0;0 1 0;0 0 1]$3x3 Transform$rad$WORLD$true$none  CGPos=[0.208531 0.0570183 -0.0276067]  CGRot=[-0.998928 -0.0462987 0;0 0 1;-0.0462987 0.998928 0]  CS0Pos=[]  CS0Rot=[]  CS1Pos=[0.208966 0.0598386 -0.0369903]  CS1Rot=[-0.998928 -0.0462987 0;0 0 1;-0.0462987 0.998928 0]  CS2Pos=[0.208549 0.192839 -0.028]  CS2Rot=[1 0 0;0 1 0;0 0 1]  CS3Pos=[0.209568 -0.0791614 -0.0499764]  CS3Rot=[1 0 0;0 1 0;0 0 1]  CS4Pos=[]  CS4Rot=[]  CS5Pos=[]  CS5Rot=[]  CS6Pos=[]  CS6Rot=[]  CS7Pos=[]  CS7Rot=[]  CS8Pos=[]  CS8Rot=[]  CS9Pos=[]  CS9Rot=[]  CS10Pos=[]  CS10Rot=[]  CS11Pos=[]  CS11Rot=[]  CS12Pos=[]  CS12Rot=[]  CS13Pos=[]  CS13Rot=[]  CS14Pos=[]  CS14Rot=[]  CS15Pos=[]  CS15Rot=[]  CS16Pos=[]  CS16Rot=[]  CS17Pos=[]  CS17Rot=[]  CS18Pos=[]  CS18Rot=[]  CS19Pos=[]  CS19Rot=[]  CS20Pos=[]  CS20Rot=[]
  Conn1 : PMIOPort  Port=1  Side=Left
  Conn2 : PMIOPort  Port=2  Side=Left
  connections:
  Support_oeufs-6/LConn1 -- Conn1/RConn1
  Support_oeufs-6/LConn2 -- Conn2/RConn1

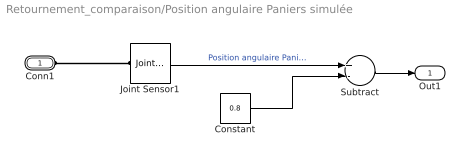
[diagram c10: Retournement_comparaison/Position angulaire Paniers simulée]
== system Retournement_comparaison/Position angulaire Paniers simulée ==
  Constant : Constant  Value=0.8
  Joint Sensor1 : mblibv1/Sensors &  Actuators/Joint Sensor  UpdateFromCAD=off  PhysicalDomain=Mechanical  PortType=blob  Muxed=on  Pose=off  Angle=on  AngleUnits=deg  ArcVelocity=off  ArcVelocityUnits=deg/s  ArcAcceleration=off  ArcAccelerationUnits=deg/s^2  CoordPosition=on  CoordPositionUnits=m  Velocity=off  VelocityUnits=m/s  Acceleration=off  AccelerationUnits=m/s^2  Quaternion=on  QuaternionDT=off  QuaternionDDT=off  QuaternionUnits=off  OutputVector=[1]  ActiveIO=on  Width=1  DialogClass=MechanicalSensorBlock  Primitive=R1  Force=off  ForceUnits=N  Torque=off  TorqueUnits=N*m  ReferenceFrame=Absolute (World)  ReactionSensedSide=Follower  ReactionReferenceFrame=Absolute (World)  ReactionForce=off  ReactionForceUnits=N  ReactionMoment=off  ReactionMomentUnits=N*m
  Subtract : Sum  Inputs=+-
  Conn1 : PMIOPort  Port=1  Side=Left
  Out1 : Outport
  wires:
  Joint Sensor1/1 -> Subtract/1  "Position angulaire Paniers simulée"
  Subtract/1 -> Out1/1
  Constant/1 -> Subtract/2
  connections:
  Joint Sensor1/LConn1 -- Conn1/RConn1

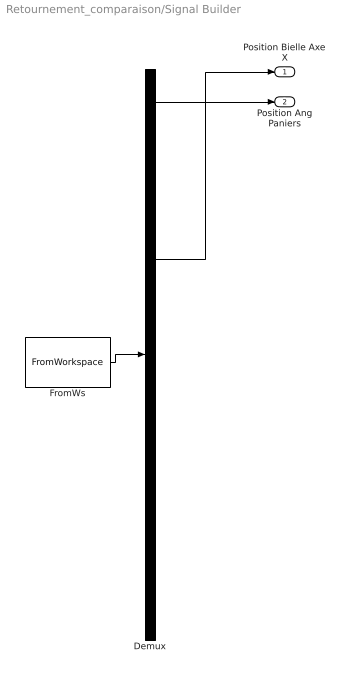
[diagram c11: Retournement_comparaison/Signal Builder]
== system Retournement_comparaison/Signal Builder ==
  Demux : Demux  Tag=STV Demux  Outputs=2
  FromWs : FromWorkspace  Tag=STV FromWs  VariableName=tuvar  SampleTime=0  OutputAfterFinalValue=Setting to zero
  Position Bielle Axe X : Outport  Tag=STV Outport
  Position Ang Paniers : Outport  Tag=STV Outport  Port=2
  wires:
  Demux/1 -> Position Bielle Axe X/1
  FromWs/1 -> Demux/1
  Demux/2 -> Position Ang Paniers/1
